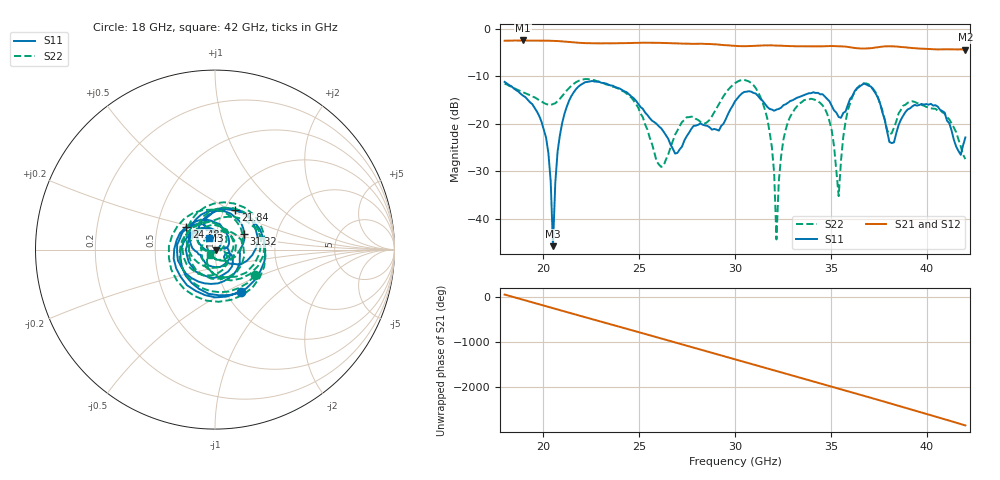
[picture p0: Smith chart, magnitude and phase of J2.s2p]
!Agilent Technologies,N5230A,US43500212,A.07.50.67
!Agilent N5230A: A.07.50.67
!Date: Monday, September 22, 2025 05:51:40
!Correction: S11(Full 2 Port(1,2))
!S21(Full 2 Port(1,2))
!S12(Full 2 Port(1,2))
!S22(Full 2 Port(1,2))
!S2P File: Measurements: S11, S21, S12, S22:
# Hz S  dB  R 50
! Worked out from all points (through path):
!   201 points, 18 GHz to 42 GHz, reference 50 ohm
!   highest |S21| = -2.40 dB at 18.96 GHz (marker M1); lowest = -4.4 dB at 42 GHz (marker M2)
!   lowest |S11| = -45.8 dB at 20.52 GHz (marker M3), VSWR 1.01, Z = 50.4 - j0.324 ohm
!   |S11| at or under -10 dB: start of sweep to end of sweep
!   |S22| runs from -44.4 to -10.5 dB; largest |S21 - S12| = 0.008
!   S11 on the Smith chart (normalised r, x): 18 GHz: 1.17, -0.60; 21.84 GHz: 1.13, +0.53; 24.48 GHz: 0.70, +0.19; 31.32 GHz: 1.36, +0.24; 42 GHz: 0.93, +0.12
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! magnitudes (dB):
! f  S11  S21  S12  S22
! 18 GHz  -11.1  -2.5  -2.5  -11.6
! 18.96 GHz  -14.1  -2.4  -2.4  -13.3
! 20.16 GHz  -22.9  -2.4  -2.4  -15.8
! 20.52 GHz  -45.8  -2.5  -2.5  -15.8
! 20.88 GHz  -22.4  -2.6  -2.6  -14.7
! 21.84 GHz  -12.2  -2.9  -2.9  -11.0
! 22.08 GHz  -11.5  -2.9  -2.9  -10.6
! 24.48 GHz  -13.8  -3.0  -3.0  -14.0
! 26.04 GHz  -20.5  -2.9  -2.9  -28.6
! 30 GHz  -15.2  -3.5  -3.5  -11.4
! 31.32 GHz  -14.7  -3.5  -3.5  -14.3
! 31.92 GHz  -17.0  -3.4  -3.4  -24.9
! 32.16 GHz  -17.0  -3.5  -3.5  -44.4
! 32.64 GHz  -15.9  -3.5  -3.5  -21.2
! 34.08 GHz  -13.3  -3.7  -3.7  -14.8
! 34.92 GHz  -15.2  -3.6  -3.6  -19.4
! 35.4 GHz  -18.6  -3.6  -3.6  -35.3
! 35.76 GHz  -17.4  -3.7  -3.7  -19.5
! 36.36 GHz  -12.5  -4.0  -4.0  -12.5
! 38.04 GHz  -23.8  -3.6  -3.6  -22.2
! 40.68 GHz  -17.0  -4.3  -4.2  -17.1
! 42 GHz  -22.9  -4.4  -4.3  -27.4
